DATA_BLOCK "DB_ALLARMI"
TITLE =
{ S7_language := '9(1) Inglese (Stati Uniti)  09.12.2014  12:08:08' }
VERSION : 0.1


  STRUCT
   D08_Q01 : BOOL ;	//S.T. ALIMENTATORI 24VDC
   SIMOTION : BOOL ;	//S.T. ALIMENTAZIONE 24VDC SIMOTION
   PLC : BOOL ;	//S.T. ALIMENTAZIONE 24VDC PLC
   CASSETTE : BOOL ;	//S.T. ALIMENTAZIONE 24VDC CASSETTE
   D10_Q01 : BOOL ;	//S.T. ALIMENTAZIONE TRAFO 115VAC
   D10_Q02 : BOOL ;	//S.T. USCITA TRAFO 115VAC
   E08_Q01 : BOOL ;	//S.T. EVACUATORE TRUCIOLI 1
   E08_S02_3 : BOOL ;	//MANCATA PARTENZA EVACUATORE TRUCIOLI 1
   E08_Q02 : BOOL ;	//S.T. EVACUATORE TRUCIOLI 2
   E08_S28_6 : BOOL ;	//MANCATA PARTENZA EVACUATORE TRUCIOLI 2
   E08_Q03 : BOOL ;	//S.T. EVACUATORE TRUCIOLI 3
   E08_S28_7 : BOOL ;	//MANCATA PARTENZA EVACUATORE TRUCIOLI 3
   E09_Q01 : BOOL ;	//S.T. CENTRALINA IDRAULICA
   E09_A01 : BOOL ;	//ALTA TEMPERATURA MOTORE CENTRALINA IDRAULICA
   E09_F01_0 : BOOL ;	//MANCANZA  PRESSIONE OLIO CENTRALINA IDRAULICA
   E09_F01_3 : BOOL ;	//INTASAMENTO FILTRO OLIO CENTRALINA IDRAULICA
   E09_S01_HH : BOOL ;	//ALTISSIMO LIVELLO OLIO CENTRALINA IDRAULICA
   E09_S01_H : BOOL ;	//ALTO LIVELLO OLIO CENTRALINA IDRAULICA
   E09_S01_L : BOOL ;	//BASSO LIVELLO OLIO CENTRALINA IDRAULICA
   E09_S01_LL : BOOL ;	//BASSISSIMO LIVELLO OLIO CENTRALINA IDRAULICA
   E09_S01_FUGA : BOOL ;	//FUGA OLIO CENTRALINA IDRAULICA
   E51_Q01 : BOOL ;	//S.T. FRESATRICE PLANETARIA 1
   E51_A01 : BOOL ;	//ALTA TEMPERATURA MOTORE FRESATRICE PLANETARIA 1
   E51_T01 : BOOL ;	//ALTA CORRENTE MOTORE FRESATRICE PLANETARIA 1
   E51_MP : BOOL ;	//MANCATA PARTENZA MOTORE FRESATRICE PLANETARIA 1
   E52_Q01 : BOOL ;	//S.T. FRESATRICE PLANETARIA 2
   E52_A01 : BOOL ;	//ALTA TEMPERATURA MOTORE FRESATRICE PLANETARIA 2
   E52_T01 : BOOL ;	//ALTA CORRENTE MOTORE FRESATRICE PLANETARIA 2
   E52_MP1 : BOOL ;	//MANCATA PARTENZA MOTORE FRESATRICE PLANETARIA 2
   E61_Q01 : BOOL ;	//S.T. POMPA LUBRIFICAZIONE 1
   E61_S11_1 : BOOL ;	//BASSO LIVELLO OLIO LUBRIFICAZIONE 1
   E61_F20_0 : BOOL ;	//MANCANZA PRESSIONE LUBRIFICAZIONE CONTROPUNTA 1
   E61_F20_1 : BOOL ;	//MANCANZA PRESSIONE LUBRIFICAZIONE GUIDA CONTROPUNTA 1
   E61_F20_2 : BOOL ;	//MANCANZA PRESSIONE LUBRIFICAZIONE SLITTA A CROCE 1
   E61_F20_3 : BOOL ;	//MANCANZA PRESSIONE LUBRIFICAZIONE GUIDA FRESATRICE 1
   E61_F20_4 : BOOL ;	//MANCANZA PRESSIONE LUBRIFICAZIONE FRESATRICE 1
   E61_F21_2 : BOOL ;	//MANCANZA PRESSIONE LUBRIFICAZIONE SERRAGGIO SUPPLEMENTARE 1
   E61_F20_5 : BOOL ;	//MANCANZA PRESSIONE LUBRIFICAZIONE CONTROPUNTA 2
   E61_F20_6 : BOOL ;	//MANCANZA PRESSIONE LUBRIFICAZIONE GUIDA CONTROPUNTA 2
   E61_F20_7 : BOOL ;	//MANCANZA PRESSIONE LUBRIFICAZIONE SLITTA A CROCE 2
   E61_F21_0 : BOOL ;	//MANCANZA PRESSIONE LUBRIFICAZIONE GUIDA FRESATRICE 2
   E61_F21_1 : BOOL ;	//MANCANZA PRESSIONE LUBRIFICAZIONE FRESATRICE 2
   E62_Q01 : BOOL ;	//S.T. POMPA LUBRIFICAZIONE 2 WG1
   E62_S17_1 : BOOL ;	//BASSO LIVELLO OLIO LUBRIFICAZIONE 2 WG1
   E62_F17_6 : BOOL ;	//INTASAMENTO FILTRO OLIO LUBRIFICAZIONE 2 WG1
   E62_F17_0 : BOOL ;	//MANCANZA PRESSIONE LUBRIFICAZIONE 2 WG1
   E62_Q02 : BOOL ;	//S.T. POMPA LUBRIFICAZIONE 2 WG2
   E62_S17_4 : BOOL ;	//BASSO LIVELLO OLIO LUBRIFICAZIONE 2 WG2
   E62_F17_7 : BOOL ;	//INTASAMENTO FILTRO OLIO LUBRIFICAZIONE 2 WG2
   E62_F17_3 : BOOL ;	//MANCANZA PRESSIONE LUBRIFICAZIONE 2 WG2
   E63_Q01 : BOOL ;	//S.T. POMPA LUBRIFICAZIONE 3
   E63_B11_4 : BOOL ;	//BASSO LIVELLO OLIO LUBRIFICAZIONE 3
   E63_F21_4 : BOOL ;	//MANCANZA LUBRIFICAZIONE 3 RIDOTTA MONTANTE 1
   E63_F21_5 : BOOL ;	//MANCANZA LUBRIFICAZIONE 3 MONTANTE 1
   E63_F21_6 : BOOL ;	//MANCANZA LUBRIFICAZIONE 3 RIDOTTA MONTANTE 2
   E63_F21_7 : BOOL ;	//MANCANZA LUBRIFICAZIONE 3 MONTANTE 2
   G17_S30_0 : BOOL ;	//MANCATA CHIUSURA PORTA DI CARICO
   G17_S30_1 : BOOL ;	//MANCATA APERTURA PORTA DI CARICO
   G50_S29_1 : BOOL ;	//CONTROPUNTA 1 NON AVANTI
   G50_S29_2 : BOOL ;	//CONTROPUNTA 1 NON INDIETRO
   G51_S13_4 : BOOL ;	//CONTROPUNTA 2 NON AVANTI
   G51_S13_5 : BOOL ;	//CONTROPUNTA 2 NON INDIETRO
   G51_F13_6 : BOOL ;	//CONTROPUNTA 2 NON AVANTI IN PRESSIONE
   G52_S12_5 : BOOL ;	//MANDRINO 1 NON BLOCCATO
   G52_S12_7 : BOOL ;	//MANDRINO 1 NON SBLOCCATO
   G52_F12_6 : BOOL ;	//MANDRINO 1 NON CHIUSO IN PRESSIONE
   G53_S29_5 : BOOL ;	//MANDRINO 2 NON BLOCCATO
   G53_S29_7 : BOOL ;	//MANDRINO 2 NON SBLOCCATO
   G53_F29_6 : BOOL ;	//MANDRINO 2 NON CHIUSO IN PRESSIONE
   G64_S27_6 : BOOL ;	//SPORTELLO TRUCIOLI 1 NON APERTO
   G64_S27_7 : BOOL ;	//SPORTELLO TRUCIOLI 1 NON CHIUSO
   G65_S07_6 : BOOL ;	//SPORTELLO TRUCIOLI 2 NON APERTO
   G65_S07_7 : BOOL ;	//SPORTELLO TRUCIOLI 2 NON CHIUSO
   G68_S14_6 : BOOL ;	//CONTROPUNTA 1 NON  DISACCOPPIATA
   G68_S14_7 : BOOL ;	//CONTROPUNTA 1 NON  ACCOPPIATA
   G68_F14_5 : BOOL ;	//CONTROPUNTA 1 NON  BLOCCATA
   G69_S14_2 : BOOL ;	//CONTROPUNTA 2 NON  DISACCOPPIATA
   G69_S14_3 : BOOL ;	//CONTROPUNTA 2 NON  ACCOPPIATA
   G69_F14_1 : BOOL ;	//CONTROPUNTA 2 NON  BLOCCATA
   G70_F15_7 : BOOL ;	//CARRO DI SERRAGGIO 1 NON BLOCCATO IN PRESSIONE
   G70_F16_0 : BOOL ;	//CARRO DI SERRAGGIO 2 NON BLOCCATO IN PRESSIONE
   G70_F16_1 : BOOL ;	//CUNEO DI SERRAGGIO NON BLOCCATO IN PRESSIONE
   G70_F16_2 : BOOL ;	//STAFFA DI SERRAGGIO NON BLOCCATA IN PRESSIONE
   G70_S15_0 : BOOL ;	//CARRO DI SERRAGGIO 1 NON BLOCCATO
   G70_S15_1 : BOOL ;	//CARRO DI SERRAGGIO 1 NON SBLOCCATO
   G70_S15_2 : BOOL ;	//CARRO DI SERRAGGIO 2 NON BLOCCATO
   G70_S15_3 : BOOL ;	//CARRO DI SERRAGGIO 2 NON SBLOCCATO
   G70_S15_4 : BOOL ;	//STAFFA DI SERRAGGIO NON BLOCCATA
   G70_S15_5 : BOOL ;	//STAFFA DI SERRAGGIO NON SBLOCCATA
   G70_S15_6 : BOOL ;	//CUNEO DI SERRAGGIO NON SBLOCCATO
   G70_F16_3 : BOOL ;	//CUNEO DI SERRAGGIO NON IN PRESSIONE
   G71_F08_3 : BOOL ;	//MANCANZA PRESSIONE ARIA MACCHINA
   G76_F28_5 : BOOL ;	//PREZZO NON PRESENTE SU PALETTA
   G77_FE28_2 : BOOL ;	//SLITTA A CROCE 1 NON SBLOCCATA
   G77_FE28_3 : BOOL ;	//SLITTA A CROCE 1 NON BLOCCATA
   G77_FE22_6 : BOOL ;	//SLITTA A CROCE 2 NON SBLOCCATA
   G77_FE22_7 : BOOL ;	//SLITTA A CROCE 2 NON BLOCCATA
   K10_S25_1 : BOOL ;	//ASSE X IN EXTRACORSA +
   K10_S25_2 : BOOL ;	//ASSE X IN EXTRACORSA -
   K10_S27_2 : BOOL ;	//ASSE X NON ABILITATO
   K10_B03 : BOOL ;	//ASSE X STRAPPO GIUNTO
   K11_S25_5 : BOOL ;	//ASSE Z IN EXTRACORSA +
   K11_S25_6 : BOOL ;	//ASSE Z IN EXTRACORSA -
   K11_B03 : BOOL ;	//ASSE Z STRAPPO GIUNTO
   K11_S27_0 : BOOL ;	//CONTROPUNTA ASSE Z IN EXTRACORSA +
   K11_S27_1 : BOOL ;	//CONTROPUNTA ASSE Z IN EXTRACORSA -
   K11_S14_4 : BOOL ;	//ST1 NON ACCOPPIATO
   K11_S27_3 : BOOL ;	//X+, C-, AUTOCENTRANTE 1 NON LIBERI
   K11_S26_0 : BOOL ;	//SELETTORE POSIZIONE WG2 SORPASSATO
   K11_S26_1 : BOOL ;	//CONTROLLO DI SICUREZZA WG1 ESPULSIONE UTENSILE
   K15_S26_3 : BOOL ;	//ASSE C IN EXTRACORSA +
   K15_S26_4 : BOOL ;	//ASSE C IN EXTRACORSA -
   K15_S26_2 : BOOL ;	//ASSE C NON ABILITATO CON ASSE Z
   K20_S05_1 : BOOL ;	//ASSE X2 IN EXTRACORSA +
   K20_S05_2 : BOOL ;	//ASSE X2 IN EXTRACORSA -
   K20_S07_2 : BOOL ;	//ASSE X2 NON ABILITATO
   K20_B03 : BOOL ;	//ASSE X2 STRAPPO GIUNTO
   K21_S05_5 : BOOL ;	//ASSE Z2 IN EXTRACORSA +
   K21_S05_6 : BOOL ;	//ASSE Z2 IN EXTRACORSA -
   K21_B03 : BOOL ;	//ASSE Z2 STRAPPO GIUNTO
   K21_S07_0 : BOOL ;	//CONTROPUNTA ASSE Z2 IN EXTRACORSA +
   K21_S07_1 : BOOL ;	//CONTROPUNTA ASSE Z2 IN EXTRACORSA -
   K21_S14_0 : BOOL ;	//ST2 NON ACCOPPIATO
   K21_S07_3 : BOOL ;	//X2+, C2-, AUTOCENTRANTE 2 NON LIBERI
   K21_S06_0 : BOOL ;	//SELETTORE POSIZIONE WG2 SORPASSATO
   K21_S06_1 : BOOL ;	//CONTROLLO DI SICUREZZA WG2 ESPULSIONE UTENSILE
   K25_S06_3 : BOOL ;	//ASSE C2 IN EXTRACORSA +
   K25_S06_4 : BOOL ;	//ASSE C2 IN EXTRACORSA -
   K25_S06_2 : BOOL ;	//ASSE C2 NON ABILITATO CON ASSE Z2
   M00_S01 : BOOL ;	//PULSANTE EMERGENZA QUADRO GENERALE PREMUTO
   M31_S01 : BOOL ;	//PULSANTE EMERGENZA PULPITO PREMUTO
   M31_S02 : BOOL ;	//CHIAVE DI SICUREZZA MACCHINA
   M31_I13 : BOOL ;	//FEEDBACK CONTATTORI EMERGENZA
   M03_S01 : BOOL ;	//PORTA 1 APERTA
   M04_S01 : BOOL ;	//PORTA 2 APERTA
   M04_S03 : BOOL ;	//PORTA 3 APERTA
   EMERGENZA : BOOL ;	//EMERGENZA MACCHINA
   spare : BOOL ;
   spare1 : BOOL ;
   spare2 : BOOL ;
   spare3 : BOOL ;
   spare4 : BOOL ;
   spare5 : BOOL ;
   spare6 : BOOL ;
   spare7 : BOOL ;
   spare8 : BOOL ;
   spare9 : BOOL ;
   spare10 : BOOL ;
   spare11 : BOOL ;
   spare12 : BOOL ;
   spare13 : BOOL ;
   spare14 : BOOL ;
   spare15 : BOOL ;
   spare16 : BOOL ;
   spare17 : BOOL ;
   spare18 : BOOL ;
   spare19 : BOOL ;
   spare20 : BOOL ;
   spare21 : BOOL ;
   spare22 : BOOL ;
  END_STRUCT ;
BEGIN
   D08_Q01 := FALSE;
   SIMOTION := FALSE;
   PLC := FALSE;
   CASSETTE := FALSE;
   D10_Q01 := FALSE;
   D10_Q02 := FALSE;
   E08_Q01 := FALSE;
   E08_S02_3 := FALSE;
   E08_Q02 := FALSE;
   E08_S28_6 := FALSE;
   E08_Q03 := FALSE;
   E08_S28_7 := FALSE;
   E09_Q01 := FALSE;
   E09_A01 := FALSE;
   E09_F01_0 := FALSE;
   E09_F01_3 := FALSE;
   E09_S01_HH := FALSE;
   E09_S01_H := FALSE;
   E09_S01_L := FALSE;
   E09_S01_LL := FALSE;
   E09_S01_FUGA := FALSE;
   E51_Q01 := FALSE;
   E51_A01 := FALSE;
   E51_T01 := FALSE;
   E51_MP := FALSE;
   E52_Q01 := TRUE;
   E52_A01 := FALSE;
   E52_T01 := FALSE;
   E52_MP1 := FALSE;
   E61_Q01 := FALSE;
   E61_S11_1 := FALSE;
   E61_F20_0 := FALSE;
   E61_F20_1 := FALSE;
   E61_F20_2 := FALSE;
   E61_F20_3 := FALSE;
   E61_F20_4 := FALSE;
   E61_F21_2 := FALSE;
   E61_F20_5 := FALSE;
   E61_F20_6 := FALSE;
   E61_F20_7 := FALSE;
   E61_F21_0 := FALSE;
   E61_F21_1 := FALSE;
   E62_Q01 := FALSE;
   E62_S17_1 := FALSE;
   E62_F17_6 := FALSE;
   E62_F17_0 := FALSE;
   E62_Q02 := FALSE;
   E62_S17_4 := FALSE;
   E62_F17_7 := FALSE;
   E62_F17_3 := FALSE;
   E63_Q01 := FALSE;
   E63_B11_4 := FALSE;
   E63_F21_4 := FALSE;
   E63_F21_5 := FALSE;
   E63_F21_6 := FALSE;
   E63_F21_7 := FALSE;
   G17_S30_0 := FALSE;
   G17_S30_1 := FALSE;
   G50_S29_1 := FALSE;
   G50_S29_2 := FALSE;
   G51_S13_4 := FALSE;
   G51_S13_5 := FALSE;
   G51_F13_6 := FALSE;
   G52_S12_5 := FALSE;
   G52_S12_7 := FALSE;
   G52_F12_6 := FALSE;
   G53_S29_5 := FALSE;
   G53_S29_7 := FALSE;
   G53_F29_6 := FALSE;
   G64_S27_6 := FALSE;
   G64_S27_7 := FALSE;
   G65_S07_6 := FALSE;
   G65_S07_7 := FALSE;
   G68_S14_6 := FALSE;
   G68_S14_7 := FALSE;
   G68_F14_5 := FALSE;
   G69_S14_2 := FALSE;
   G69_S14_3 := FALSE;
   G69_F14_1 := FALSE;
   G70_F15_7 := FALSE;
   G70_F16_0 := FALSE;
   G70_F16_1 := FALSE;
   G70_F16_2 := FALSE;
   G70_S15_0 := FALSE;
   G70_S15_1 := FALSE;
   G70_S15_2 := FALSE;
   G70_S15_3 := FALSE;
   G70_S15_4 := FALSE;
   G70_S15_5 := FALSE;
   G70_S15_6 := FALSE;
   G70_F16_3 := FALSE;
   G71_F08_3 := FALSE;
   G76_F28_5 := FALSE;
   G77_FE28_2 := FALSE;
   G77_FE28_3 := FALSE;
   G77_FE22_6 := FALSE;
   G77_FE22_7 := FALSE;
   K10_S25_1 := FALSE;
   K10_S25_2 := FALSE;
   K10_S27_2 := FALSE;
   K10_B03 := FALSE;
   K11_S25_5 := FALSE;
   K11_S25_6 := FALSE;
   K11_B03 := FALSE;
   K11_S27_0 := FALSE;
   K11_S27_1 := FALSE;
   K11_S14_4 := FALSE;
   K11_S27_3 := FALSE;
   K11_S26_0 := FALSE;
   K11_S26_1 := FALSE;
   K15_S26_3 := FALSE;
   K15_S26_4 := FALSE;
   K15_S26_2 := FALSE;
   K20_S05_1 := FALSE;
   K20_S05_2 := FALSE;
   K20_S07_2 := FALSE;
   K20_B03 := FALSE;
   K21_S05_5 := FALSE;
   K21_S05_6 := FALSE;
   K21_B03 := FALSE;
   K21_S07_0 := FALSE;
   K21_S07_1 := FALSE;
   K21_S14_0 := FALSE;
   K21_S07_3 := FALSE;
   K21_S06_0 := FALSE;
   K21_S06_1 := FALSE;
   K25_S06_3 := FALSE;
   K25_S06_4 := FALSE;
   K25_S06_2 := FALSE;
   M00_S01 := FALSE;
   M31_S01 := FALSE;
   M31_S02 := FALSE;
   M31_I13 := FALSE;
   M03_S01 := FALSE;
   M04_S01 := FALSE;
   M04_S03 := FALSE;
   EMERGENZA := FALSE;
   spare := FALSE;
   spare1 := FALSE;
   spare2 := FALSE;
   spare3 := FALSE;
   spare4 := FALSE;
   spare5 := FALSE;
   spare6 := FALSE;
   spare7 := FALSE;
   spare8 := FALSE;
   spare9 := FALSE;
   spare10 := FALSE;
   spare11 := FALSE;
   spare12 := FALSE;
   spare13 := FALSE;
   spare14 := FALSE;
   spare15 := FALSE;
   spare16 := FALSE;
   spare17 := FALSE;
   spare18 := FALSE;
   spare19 := FALSE;
   spare20 := FALSE;
   spare21 := FALSE;
   spare22 := FALSE;
END_DATA_BLOCK

